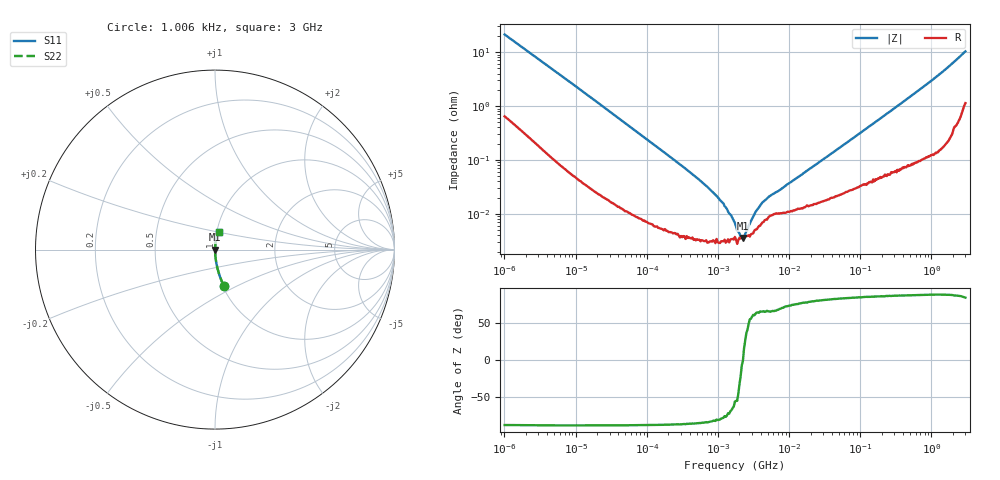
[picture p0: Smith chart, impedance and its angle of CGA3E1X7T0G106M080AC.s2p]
! S-Parameter Data Generated by TDK Corporation
! Copyright(C) 2024 TDK Corporation.
! All Rights Reserved.
! TDK P/N: CGA3E1X7T0G106M080AC (Multilayer Ceramic Chip Capacitor)
! Property: C=10uF
! Size(LxWxT): 1.6x0.8x0.8mm
! Model Type: s2p (Touchstone File Format Version 1.0)
! Frequency: DC=Yes Start=0.00100604MHz Stop=3000MHz 480points Log-sweep
! Model Generated on May 28, 2024
! Terms and conditions regarding TDK Simulation Models:
! 1)This simulation model is being provided solely for informational
!  purposes. Please refer to the specifications of the products in
!  terms of detailed characteristics of such products.
! 2)In no event shall TDK Corporation of any of its subsidiaries be
!  liable for any loss or damage arising, directly or indirectly,
!  from any information contained in this simulation model, including,
!  but not limited to loss or damages arising from any inaccuracies,
!  omissions or errors in connection with such information.
! 3)Any and all copyrights on this simulation model are owned by
!  TDK Corporation.  Duplication or redistribution of this simulation
!  model without prior written permission from TDK Corporation
!  is prohibited.
! 4)This simulation model is subject to any modification or change
!  without any prior notice.
! 5)Neither TDK Corporation nor any of its subsidiaries shall make any
!  warranty, express or implied, including but not limited to the
!  correctness, implied warranties of merchantability and fitness for
!  a particular purpose with respect to this simulation models.
! 6)The use of this simulation model shall be deemed to have consented
!  to the terms and conditions hereof.
! Port Assignments:
!  1 ---| |--- 2
! Applicable Conditions:
!  Temperature = 25 degC
!  DC Bias Voltage = 0 V
!  Small Signal Operation
# Hz S MA R 50
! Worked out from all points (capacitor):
!   479 points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, 1.006 kHz to 3 GHz, reference 50 ohm
!   read as one part in series: C = 7.36 uF near 1.083 kHz
!   lowest |Z| = 3.57 mohm at 2.244 MHz (marker M1)
!   series resonance near 2.252 MHz, so ESL is about 680 pH
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1006.04  0.2066 -76.3  0.9722 11.9  0.9722 11.9  0.2066 -76.3
1754.24  0.1235 -81.3  0.989 7.1  0.989 7.1  0.1235 -81.3
2947.59  0.0757 -84.3  0.9953 4.3  0.9953 4.3  0.0757 -84.3
12511.3  0.01874 -87.8  0.9995 1.1  0.9995 1.1  0.01874 -87.8
149930  0.001621 -88.0  0.9999 0.1  0.9999 0.1  0.001621 -88.0
364964  0.0006595 -86.6  1 0.0  1 0.0  0.0006595 -86.6
660424  0.000343 -84.8  1 0.0  1 0.0  0.000343 -84.8
888402  0.0002369 -82.4  1 0.0  1 0.0  0.0002369 -82.4
1109680  0.0001718 -79.6  1 0.0  1 0.0  0.0001718 -79.6
1386080  0.000111 -72.4  1 0.0  1 0.0  0.000111 -72.4
1492750  9.724e-05 -69.9  1 0.0  1 0.0  9.724e-05 -69.9
1796710  5.84e-05 -55.8  1 0.0  1 0.0  5.84e-05 -55.8
2244230  3.572e-05 -1.7  1 0.0  1 0.0  3.572e-05 -1.7
3018940  8.063e-05 58.0  1 -0.0  1 -0.0  8.063e-05 58.0
3251260  9.771e-05 59.9  1 -0.0  1 -0.0  9.771e-05 59.9
4214440  0.0001629 64.9  0.9999 -0.0  0.9999 -0.0  0.0001629 64.9
5264160  0.0002109 65.0  0.9999 -0.0  0.9999 -0.0  0.0002109 65.0
7626280  0.0002841 68.7  0.9999 -0.0  0.9999 -0.0  0.0002841 68.7
2.15311e7  0.0007489 78.8  0.9999 -0.0  0.9999 -0.0  0.0007489 78.8
2.50734e8  0.007612 85.5  0.9994 -0.4  0.9994 -0.4  0.007612 85.5
1.19468e9  0.03541 85.8  0.998 -2.0  0.998 -2.0  0.03541 85.8
3e9  0.1017 77.9  0.9837 -5.8  0.9837 -5.8  0.1017 77.9
